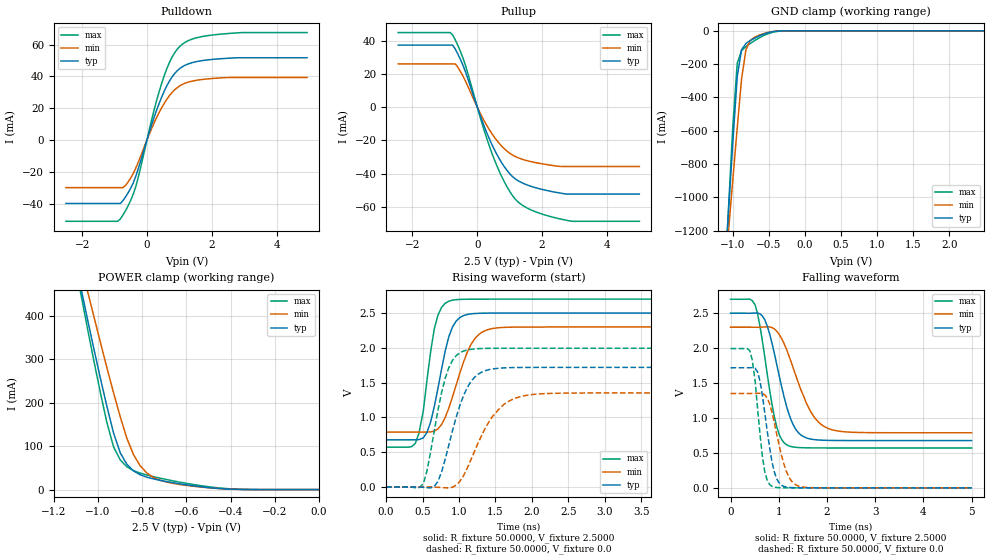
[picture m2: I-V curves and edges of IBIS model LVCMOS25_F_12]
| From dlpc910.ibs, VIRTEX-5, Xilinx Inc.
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|   Model LVCMOS25_F_12
[Model]  LVCMOS25_F_12
Model_type I/O
Polarity   Non-Inverting
Enable   Active-Low
Vinl = 0.65
Vinh = 1.85
Vmeas =  1.2500V
Cref =   0.0F
Rref =   1.0000M
Vref =   0.0V
C_comp   6.0000pF   6.0000pF   6.0000pF
[Model Spec]
Vinl   0.65   0.6   0.7
Vinh   1.85   1.7   2.0
[Temperature Range]   25.0000   85.0000   0.0
[Voltage Range]   2.5000V   2.3000V   2.7000V
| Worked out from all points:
|   slope of the pulldown table from 0 to 0.375 V, typ, clamps not added: 16.3 ohm
|   slope of the pullup table from 0 to 0.375 V, typ, clamps not added: 19.5 ohm
|   GND clamp passes 1 mA (typ) near -0.35 V on its own axis
|   POWER clamp passes 1 mA (typ) near -0.40 V on its own axis
|   rising waveform, R_fixture 50.0000, V_fixture 2.5000: 20-80 % time 219ps typ, 297ps min, 169ps max; typ from 0.677 V to 2.5 V
|   rising waveform, R_fixture 50.0000, V_fixture 0.0: 20-80 % time 294ps typ, 403ps min, 230ps max; typ from 0 V to 1.72 V
|   falling waveform, R_fixture 50.0000, V_fixture 2.5000: 20-80 % time 383ps typ, 512ps min, 296ps max; typ from 2.5 V to 0.677 V
|   falling waveform, R_fixture 50.0000, V_fixture 0.0: 20-80 % time 222ps typ, 282ps min, 176ps max; typ from 1.72 V to 0 V
[Pulldown]
|Voltage   I(typ)   I(min)   I(max)
-2.5V     -39.8mA    -29.84mA   -51mA
-900mV    -39.8mA    -29.84mA   -51mA
-820mV    -39.8mA    -29.84mA   -49.53mA
-660mV    -35.7mA    -28.49mA   -44.35mA
-340mV    -22.55mA   -17.45mA   -28.94mA
220mV     14.2mA     10.7mA     18.76mA
540mV     30.98mA    23.3mA     40.82mA
780mV     39.81mA    30.03mA    52.29mA
1.1V      46.18mA    35.06mA    60.36mA
1.5V      49.17mA    37.49mA    64.12mA
2.22V     51.04mA    39.01mA    66.47mA
4.94V     51.73mA    39.36mA    67.56mA
[Pullup]
|Voltage   I(typ)   I(min)   I(max)
-2.44V    37.46mA    26.15mA    45.04mA
-840mV    37.46mA    26.15mA    45.04mA
-760mV    37.46mA    26.15mA    43.62mA
-600mV    32.11mA    24.14mA    37.29mA
-360mV    21.09mA    15.58mA    24.96mA
120mV     -6.701mA   -4.795mA   -8.164mA
520mV     -25.32mA   -17.91mA   -31.29mA
920mV     -38.23mA   -26.59mA   -48.16mA
1.32V     -45.02mA   -30.95mA   -58.15mA
1.96V     -49.41mA   -34.03mA   -64.25mA
2.92V     -52.44mA   -35.78mA   -68.84mA
5V        -52.44mA   -35.78mA   -68.84mA
[GND_clamp]
|Voltage   I(typ)   I(min)   I(max)
-2.5V     -11.29A    -8.704A    -13.53A
-1.12V    -1.497A    -1.51A     -1.57A
-1.06V    -1.075A    -1.198A    -1.059A
-1V       -662mA     -888.5mA   -563.2mA
-940mV    -273.6mA   -582.9mA   -195.1mA
-880mV    -113.7mA   -290.3mA   -119.7mA
-820mV    -76.4mA    -115.2mA   -95.07mA
-760mV    -58.66mA   -58.46mA   -76.31mA
-700mV    -44.35mA   -38.35mA   -59.24mA
-520mV    -12.14mA   -10.32mA   -18.61mA
-340mV    -602.1uA   -638.4uA   -1.401mA
2.48V     19.95nA    6.298uA    40.3nA
[POWER_clamp]
|Voltage   I(typ)   I(min)   I(max)
-2.49V    3.897A     3.398A     4.279A
-1.08V    470.7mA    523.2mA    456.9mA
-1.05V    398.2mA    462.2mA    377.2mA
-1.02V    327.1mA    401.4mA    299.7mA
-960mV    191.8mA    281.1mA    154.7mA
-930mV    130.6mA    223.5mA    98.93mA
-900mV    85.26mA    168.6mA    68.69mA
-840mV    43.25mA    81.1mA     43.8mA
-780mV    28.81mA    38.65mA    33.69mA
-690mV    18.53mA    17.37mA    23.2mA
-540mV    6.864mA    6.149mA    9.448mA
0V        21.48nA    108.1nA    47.01nA
[Ramp]
| variable   typ   min   max
dV/dt_r  1.0314/0.2914n   0.8106/0.3977n   1.1964/0.2261n
dV/dt_f  1.0938/0.3812n   0.9067/0.5107n   1.2773/0.2941n
R_load = 50.0000
[Rising Waveform]
R_fixture= 50.0000
V_fixture= 2.5000
V_fixture_min= 2.3000
V_fixture_max= 2.7000
|time   V(typ)   V(min)   V(max)
0s        676.9mV    788.8mV    571.1mV
400ps     677mV      788.8mV    625.3mV
510ps     705.3mV    788.7mV    1.093V
660ps     1.152V     802.3mV    2.27V
760ps     1.692V     896.4mV    2.581V
860ps     2.16V      1.134V     2.67V
960ps     2.384V     1.464V     2.692V
1.16ns    2.488V     2.04V      2.699V
1.41ns    2.499V     2.266V     2.7V
5ns       2.5V       2.3V       2.7V
[Rising Waveform]
R_fixture= 50.0000
V_fixture= 0.0
|time   V(typ)   V(min)   V(max)
0s        0V         672.7nV    0V
510ps     -5.436mV   16.3uV     45.73mV
660ps     7.27mV     -2.544mV   806.5mV
810ps     397.3mV    -12.29mV   1.561V
910ps     807.9mV    -3.987mV   1.82V
1.06ns    1.308V     158.5mV    1.953V
1.21ns    1.574V     505.7mV    1.984V
1.46ns    1.696V     1.013V     1.993V
1.82ns    1.717V     1.292V     1.994V
5ns       1.719V     1.351V     1.994V
[Falling Waveform]
R_fixture= 50.0000
V_fixture= 2.5000
V_fixture_min= 2.3000
V_fixture_max= 2.7000
|time   V(typ)   V(min)   V(max)
0s        2.5V       2.3V       2.7V
510ps     2.503V     2.299V     2.618V
710ps     2.406V     2.304V     1.871V
910ps     1.918V     2.274V     1.012V
1.01ns    1.6V       2.194V     762.1mV
1.16ns    1.171V     1.983V     617.4mV
1.46ns    756mV      1.402V     575.5mV
1.72ns    691.9mV    1.028V     572mV
2.02ns    679.8mV    851.5mV    571.2mV
5ns       677mV      788.8mV    571.1mV
[Falling Waveform]
R_fixture= 50.0000
V_fixture= 0.0
|time   V(typ)   V(min)   V(max)
0s        1.719V     1.351V     1.994V
400ps     1.72V      1.351V     1.961V
510ps     1.71V      1.351V     1.527V
610ps     1.53V      1.354V     772.9mV
710ps     1.071V     1.332V     229.4mV
860ps     371.1mV    1.077V     21.38mV
960ps     125.2mV    758.3mV    5.018mV
1.16ns    10.78mV    231.4mV    794.4uV
1.41ns    1.251mV    25.62mV    191.2uV
5ns       50.28uV    48.02uV    15.72uV
